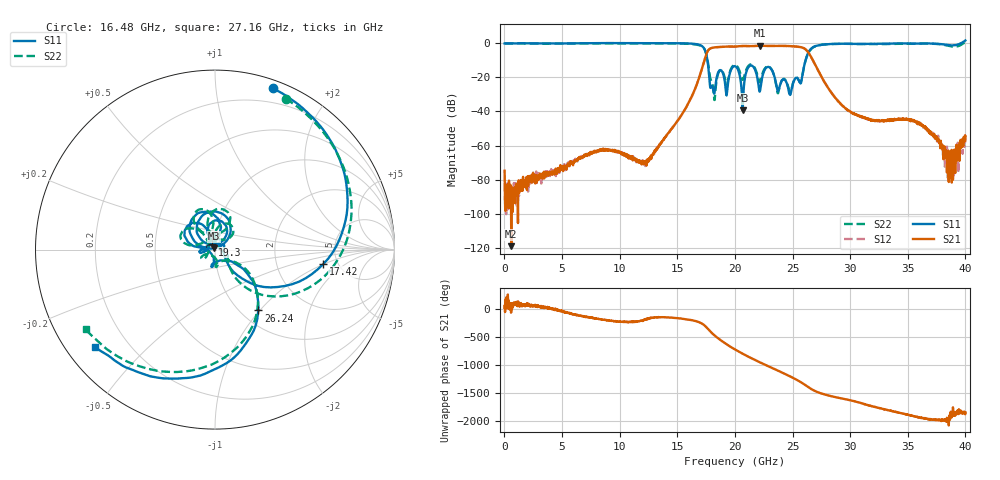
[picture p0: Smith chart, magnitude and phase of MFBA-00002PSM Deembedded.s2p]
!Keysight Technologies,N5247B,US58420632,A.15.75.19
!Date: Thursday, September 22, 2022 16:06:54
!Correction: S11(C  2-Port  )
!S41(C  2-Port  )
!S14(C  2-Port  )
!S44(C  2-Port  )
!S2P File: Measurements: S11, S41, S14, S44:
# Hz S  dB  R 50
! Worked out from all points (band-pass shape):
!   2000 points, 20 MHz to 40 GHz, reference 50 ohm
!   highest |S21| = -1.48 dB at 22.16 GHz (marker M1); lowest = -119.0 dB at 600 MHz (marker M2)
!   |S21| within 3 dB of the highest: 17.65 GHz to 26.26 GHz (8.604 GHz wide, 39.2 % of centre)
!   lowest |S11| = -39.4 dB at 20.68 GHz (marker M3), VSWR 1.02, Z = 49.3 + j0.767 ohm
!   |S11| at or under -10 dB: 17.62 GHz to 26.13 GHz (8.512 GHz wide, 38.9 % of centre)
!   |S22| runs from -33.3 to 0.6 dB; largest |S21 - S12| = 0.0018
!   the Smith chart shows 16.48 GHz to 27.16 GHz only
!   S11 on the Smith chart (normalised r, x): 16.48 GHz: 0.07, +1.42; 17.42 GHz: 3.84, -0.98; 19.3 GHz: 0.97, +0.06; 26.24 GHz: 1.20, -0.98; 27.16 GHz: 0.09, -0.35
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2e7  -0.16 -0.4  -74.73 16.3  -81.99 107.1  -0.12 -0.4
6e8  -0.09 -7.8  -118.95 -39.3  -89.95 146.4  -0.20 -8.4
6.7e9  -0.05 -98.7  -66.80 -131.2  -66.28 -128.7  -0.07 -101.7
1.336e10  -0.02 140.3  -60.72 -155.1  -60.78 -153.5  -0.15 135.6
1.648e10  -0.40 70.4  -27.86 143.6  -27.86 143.7  -0.64 65.0
1.742e10  -4.31 -7.6  -8.43 49.8  -8.43 49.8  -4.32 -16.4
1.814e10  -28.02 45.1  -2.54 -101.5  -2.54 -101.4  -27.67 -10.7
1.866e10  -15.94 92.6  -2.25 173.3  -2.26 173.4  -16.30 70.3
1.93e10  -29.87 117.0  -1.95 82.2  -1.96 82.2  -24.19 77.5
2.002e10  -13.50 88.0  -1.98 -8.4  -1.99 -8.4  -12.82 78.5
2.068e10  -39.43 133.3  -1.64 -83.8  -1.64 -83.8  -21.43 95.6
2.216e10  -28.36 128.7  -1.48 124.5  -1.49 124.5  -22.86 137.2
2.338e10  -18.45 110.7  -1.55 9.5  -1.57 9.4  -18.43 127.3
2.44e10  -21.93 -178.8  -1.62 -87.9  -1.62 -87.9  -21.61 -152.2
2.532e10  -20.34 -99.3  -1.95 177.5  -1.96 177.5  -20.17 -85.3
2.624e10  -7.62 -54.5  -4.33 59.8  -4.33 59.8  -7.90 -54.0
2.668e10  -2.80 -100.4  -8.90 1.9  -8.90 1.9  -3.04 -105.1
2.716e10  -1.32 -141.0  -15.21 -45.1  -15.21 -45.2  -1.45 -148.3
2.966e10  -0.30 119.7  -38.66 -176.9  -38.62 -175.6  -0.37 118.6
3.334e10  -0.22 43.7  -45.36 -10.1  -45.18 -8.0  -0.48 44.8
3.874e10  -1.27 3.5  -65.97 -34.2  -75.71 50.1  -1.83 12.3
4e10  1.60 -18.5  -56.36 -46.8  -54.03 -55.1  0.63 -20.0
